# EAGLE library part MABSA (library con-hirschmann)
Dual SWITCH
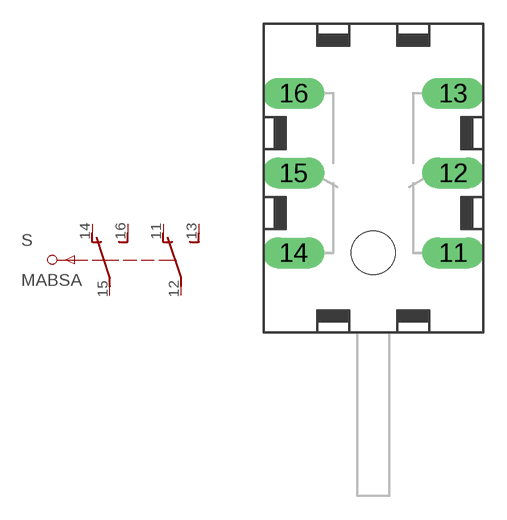
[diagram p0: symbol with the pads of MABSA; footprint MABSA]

Designator prefix S

## MABSA (OC_FARNELL: unknown; OC_NEWARK: unknown)  [MABSA]
11  11  pas
12  12  pas
13  13  pas
14  14  pas
15  15  pas
16  16  pas

## Footprint MABSA (pad centres in mm)
Dual SWITCH
drill 1.321 long: 11 5.08,-5.08; 12 5.08,0; 13 5.08,5.08; 14 -5.08,-5.08; 15 -5.08,0; 16 -5.08,5.08
hole 2.794 at 0,-5.08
